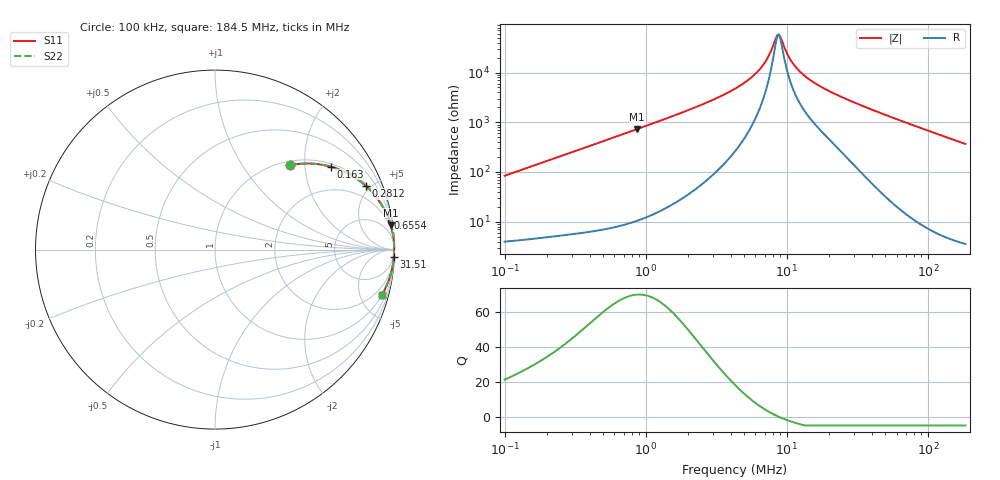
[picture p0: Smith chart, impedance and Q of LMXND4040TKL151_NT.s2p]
! LMXND4040TKL151_NT  S-PARAMETER MODEL  ( Standard Model )
! Model Generated by TAIYO YUDEN Corporation (https://www.yuden.co.jp/en/)
! Version 1.0
! TAIYO YUDEN Control No. 20251120
! Copyright(c) 2025 TAIYO YUDEN CO.,LTD. All Rights Reserved.
! Product Description (link to TY-COMPAS)
! https://ds.yuden.co.jp/TYCOMPAS/or/detail?pn=LMXND4040TKL151MNT&u=M
! Products Name : Inductors
! Characteristics :
!  Inductance : 150 [uH] , SRF(min) : 5.5 [MHz] , DC Resistance(max) : 2.76 [Ohm]
!  Rated Current : Saturation  340 [mA] , Temp Rise  380 [mA] (40 [degC])
!  Case Size : 4.0 x 4.0 / 0.157 x 0.157 [mm/inch] , Thickness : 1.8 / 0.071 [mm/inch]
!  (Conditions: Temperature = 25 [degC] , DC Bias Current = 0 [A])
! External Node Assignments :
!  1  o---GGG---o  2
! GND o---------o GND
! Frequency Range : 0.1MHz  -  184.468258MHz  [ 402 STEP ]
# MHz S RI R 50
! Freq[MHz].  S11 Real  S11 Imag  S21 Real  S21 Imag  S12 Real  S12 Imag  S22 Real  S22 Imag
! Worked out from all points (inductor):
!   401 points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, 100 kHz to 184.5 MHz, reference 50 ohm
!   read as one part in series: L = 133 uH near 103.8 kHz
!   highest Q = 69.6 at 868.9 kHz (marker M1), where L = 133 uH
!   self-resonance near 8.611 MHz
!   S11 on the Smith chart (normalised r, x): 100 kHz: 1.08, +1.68; 163 kHz: 1.09, +2.72; 281.2 kHz: 1.11, +4.68; 655.4 kHz: 1, +11; 31.51 MHz: 3, -47; 184.5 MHz: 1.07, -7.32
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0.1  0.4177 0.4701  0.5823 -0.4701  0.5823 -0.4701  0.4177 0.4701
0.163037  0.6455 0.4619  0.3545 -0.4619  0.3545 -0.4619  0.6455 0.4619
0.281232  0.8401 0.355  0.1599 -0.355  0.1599 -0.355  0.8401 0.355
0.352405  0.891 0.3017  0.109 -0.3017  0.109 -0.3017  0.891 0.3017
0.655361  0.9651 0.1761  0.0349 -0.1761  0.0349 -0.1761  0.9651 0.1761
0.868865  0.9796 0.1344  0.0204 -0.1344  0.0204 -0.1344  0.9796 0.1344
1.241892  0.9896 0.0941  0.0104 -0.0941  0.0104 -0.0941  0.9896 0.0941
2.68436  0.9973 0.0405  0.00274 -0.0405  0.00274 -0.0405  0.9973 0.0405
4.294977  0.9984 0.0211  0.00161 -0.0211  0.00161 -0.0211  0.9984 0.0211
5.484074  0.9985 0.0132  0.00146 -0.0132  0.00146 -0.0132  0.9985 0.0132
6.49511  0.9985 0.00817  0.00147 -0.00817  0.00147 -0.00817  0.9985 0.00817
7.408668  0.9985 0.00449  0.00154 -0.00449  0.00154 -0.00449  0.9985 0.00449
8.450721  0.9983 0.000917  0.00167 -0.000917  0.00167 -0.000917  0.9983 0.000917
8.77452  0.9983 -8.98e-05  0.00171 8.98e-05  0.00171 8.98e-05  0.9983 -8.98e-05
9.110726  0.9982 -0.00109  0.00176 0.00109  0.00176 0.00109  0.9982 -0.00109
10.19863  0.9981 -0.00409  0.00193 0.00409  0.00193 0.00409  0.9981 -0.00409
11.20381  0.9979 -0.00659  0.00209 0.00659  0.00209 0.00659  0.9979 -0.00659
12.77966  0.9977 -0.0101  0.00233 0.0101  0.00233 0.0101  0.9977 -0.0101
15.13571  0.9974 -0.0149  0.00264 0.0149  0.00264 0.0149  0.9974 -0.0149
31.50867  0.9961 -0.042  0.00389 0.042  0.00389 0.042  0.9961 -0.042
53.33896  0.9927 -0.0756  0.00732 0.0756  0.00732 0.0756  0.9927 -0.0756
184.4683  0.9284 -0.253  0.0716 0.253  0.0716 0.253  0.9284 -0.253
